(* Logix 5000 AddOnInstructionDefinition export AMCI_3601_AOP_Encoder_Follower; software revision 20.03 *)

ADD_ON_INSTRUCTION AMCI_3601_AOP_Encoder_Follower   (* revision 0.0, vendor AMCI, ExecuteEnableInFalse *)
// Revision note:
// 3/2020: Version 0 is the initial release
VAR_INPUT
   Axis_Status_Bits : INT; {required}
   _0_same_1_opposite_direction : BOOL;
   _0_normal_1_S_Curve_Acceleration : BOOL;
   _0_Triangular_1_Trapezoidal_S_Curve : BOOL;
   Multiplier : INT; {required}
   Divisor : INT; {required}
   Acceleration : INT; {required}
   Deceleration : INT; {required}
END_VAR
VAR_OUTPUT
   EN : BOOL; {access Read Only, visible}
   Encoder_Follower_Occurring : BOOL; {access Read Only, visible}
   ER : BOOL; {access Read Only, visible}
END_VAR
VAR_IN_OUT
   AMCI_3601_output_data : AM:1769_3601:O:0; {required}
END_VAR
VAR
   Upper_Result_X_1000 : DINT;
   command_data_block : INT[10];
        [0]   // Command Bits MSW
        [1]   // Command Bits LSW
        [2]   // Upper Target Position
        [3]   // Lower Target Position
        [4]   // Upper Programmed Speed
        [5]   // Lower Programmed Speed
END_VAR

ROUTINE EnableInFalse   (* ladder *)
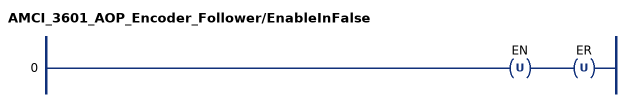
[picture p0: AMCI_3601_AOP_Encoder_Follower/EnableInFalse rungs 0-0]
   0: OTU(EN)OTU(ER);
END_ROUTINE

ROUTINE Logic   (* ladder *)
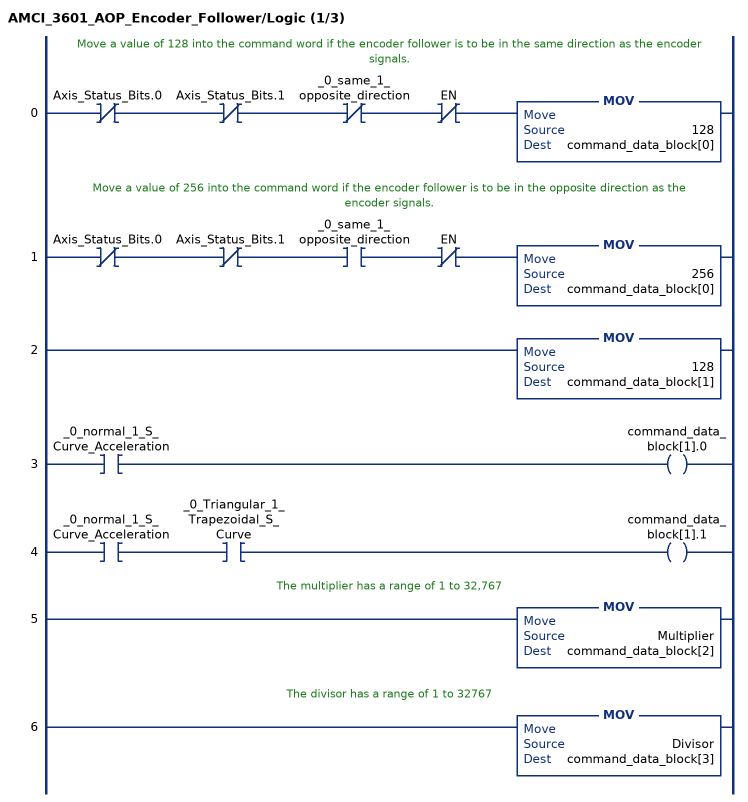
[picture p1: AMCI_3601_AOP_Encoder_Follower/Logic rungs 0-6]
   // Move a value of 128 into the command word if the encoder follower is to be in the same direction as the encoder signals.
   0: XIO(Axis_Status_Bits.0)XIO(Axis_Status_Bits.1)XIO(_0_same_1_opposite_direction)XIO(EN)MOV(128,command_data_block[0]);
   // Move a value of 256 into the command word if the encoder follower is to be in the opposite direction as the encoder signals.
   1: XIO(Axis_Status_Bits.0)XIO(Axis_Status_Bits.1)XIC(_0_same_1_opposite_direction)XIO(EN)MOV(256,command_data_block[0]);
   2: MOV(128,command_data_block[1]);
   3: XIC(_0_normal_1_S_Curve_Acceleration)OTE(command_data_block[1].0);
   4: XIC(_0_normal_1_S_Curve_Acceleration)XIC(_0_Triangular_1_Trapezoidal_S_Curve)OTE(command_data_block[1].1);
   // The multiplier has a range of 1 to 32,767
   5: MOV(Multiplier,command_data_block[2]);
   // The divisor has a range of 1 to 32767
   6: MOV(Divisor,command_data_block[3]);
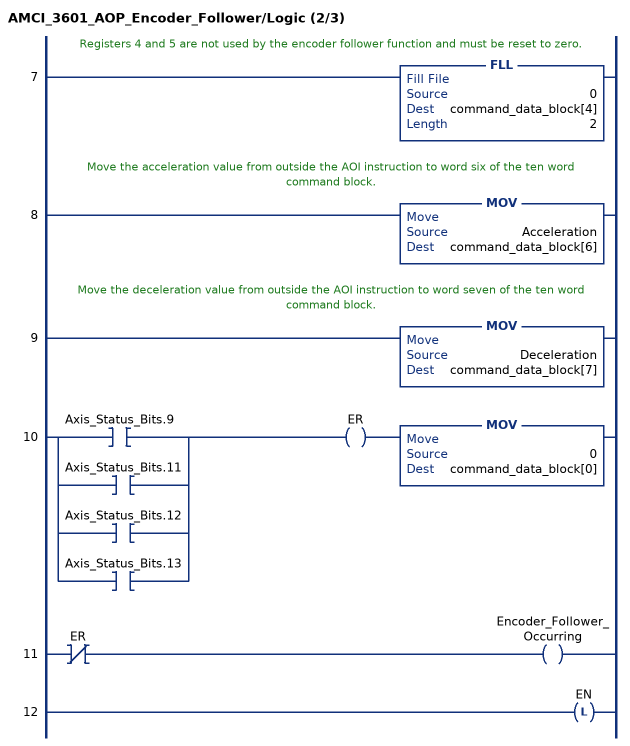
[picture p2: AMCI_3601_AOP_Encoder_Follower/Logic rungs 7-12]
   // Registers 4 and 5 are not used by the encoder follower function and must be reset to zero.
   7: FLL(0,command_data_block[4],2);
   // Move the acceleration value from outside the AOI instruction to word six of the ten word command block.
   8: MOV(Acceleration,command_data_block[6]);
   // Move the deceleration value from outside the AOI instruction to word seven of the ten word command block.
   9: MOV(Deceleration,command_data_block[7]);
   10: [XIC(Axis_Status_Bits.9) ,XIC(Axis_Status_Bits.11) ,XIC(Axis_Status_Bits.12) ,XIC(Axis_Status_Bits.13) ]OTE(ER)MOV(0,command_data_block[0]);
   11: XIO(ER)OTE(Encoder_Follower_Occurring);
   12: OTL(EN);
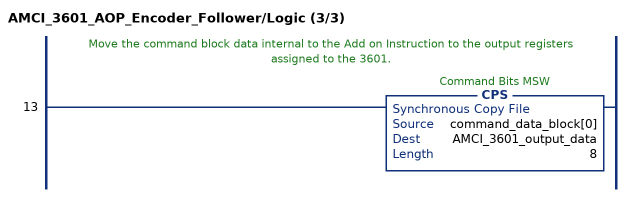
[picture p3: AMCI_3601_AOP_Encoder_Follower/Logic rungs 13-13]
   // Move the command block data internal to the Add on Instruction to the output registers assigned to the 3601.
   13: CPS(command_data_block[0],AMCI_3601_output_data,8);
END_ROUTINE
END_ADD_ON_INSTRUCTION
